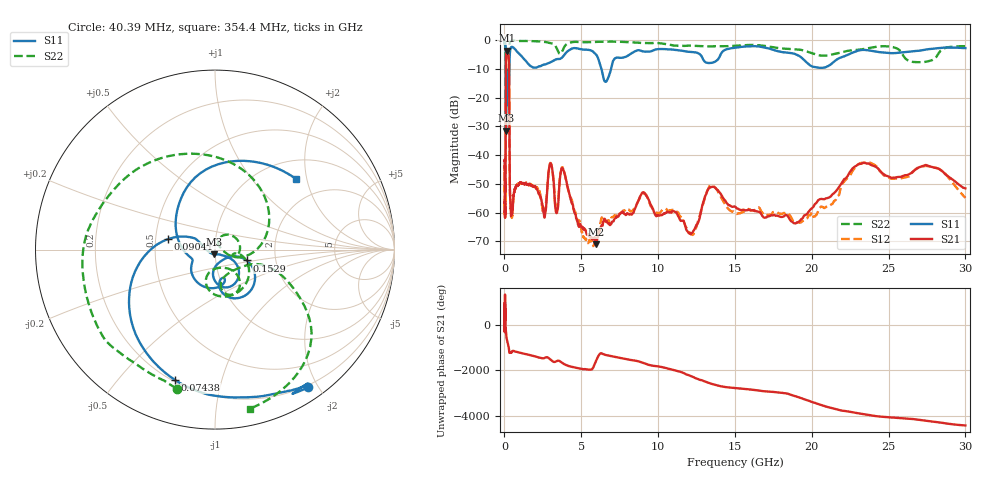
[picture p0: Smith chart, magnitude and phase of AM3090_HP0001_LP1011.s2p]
! Date/Time: Thu, Feb 28, 2019 1:54 PM
! Network Analyzer: Agilent Technologies E8364B Rev: A.07.50.67
! Sweep from 0.010 to 30.000 GHz, 1601 Points, Sweep Type: LOG
! Power Supply: 5.022 V, 0.002 A
# Hz S DB R 50
!freq MagS11 AngS11 MagS21 AngS21 MagS12 AngS12 MagS22 AngS22
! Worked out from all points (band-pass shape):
!   1601 points, 10 MHz to 30 GHz, reference 50 ohm
!   highest |S21| = -3.71 dB at 150.6 MHz (marker M1); lowest = -71.0 dB at 5.959 GHz (marker M2)
!   |S21| within 3 dB of the highest: 100.5 MHz to 284.1 MHz (183.5 MHz wide, 95.4 % of centre)
!   lowest |S11| = -31.5 dB at 98.93 MHz (marker M3), VSWR 1.05, Z = 49.6 - j2.61 ohm
!   |S11| at or under -10 dB: 89.6 MHz to 314.4 MHz (224.8 MHz wide, 111 % of centre); 6.309 GHz to 6.936 GHz (627.2 MHz wide, 9.47 % of centre)
!   |S22| runs from -30.4 to -0.2 dB; largest |S21 - S12| = 0.012
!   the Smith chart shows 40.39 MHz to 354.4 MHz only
!   S11 on the Smith chart (normalised r, x): 40.39 MHz: 0.17, -1.87; 74.38 MHz: 0.21, -0.72; 90.41 MHz: 0.58, +0.07; 152.9 MHz: 1.42, -0.18; 354.4 MHz: 1.40, +1.72
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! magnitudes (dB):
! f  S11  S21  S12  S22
! 10 MHz  -0.2  -42.0  -45.6  -0.6
! 38.04 MHz  -0.5  -58.5  -61.6  -1.7
! 40.39 MHz  -0.7  -60.8  -61.4  -1.9
! 74.38 MHz  -2.4  -47.6  -46.1  -4.4
! 90.41 MHz  -11.5  -14.9  -14.9  -11.7
! 98.93 MHz  -31.5  -7.2  -7.2  -29.8
! 115 MHz  -13.3  -4.8  -4.8  -18.4
! 144.7 MHz  -20.2  -3.8  -3.7  -19.3
! 150.6 MHz  -15.8  -3.7  -3.7  -17.3
! 152.9 MHz  -14.6  -3.7  -3.7  -16.5
! 288.7 MHz  -16.3  -7.4  -7.3  -15.4
! 354.4 MHz  -4.5  -52.2  -52.4  -0.8
! 550.5 MHz  -2.6  -57.5  -57.2  -0.3
! 2.084 GHz  -9.6  -51.6  -51.3  -0.5
! 2.61 GHz  -8.6  -61.7  -60.0  -0.6
! 3.017 GHz  -7.7  -43.0  -42.9  -1.1
! 3.385 GHz  -6.7  -60.2  -59.3  -2.7
! 3.817 GHz  -5.7  -44.8  -44.5  -3.3
! 5.959 GHz  -5.1  -71.0  -68.8  -0.7
! 7.926 GHz  -5.8  -60.8  -58.9  -0.7
! 23.48 GHz  -3.5  -42.8  -42.6  -3.0
! 30 GHz  -2.8  -51.6  -54.9  -2.2
